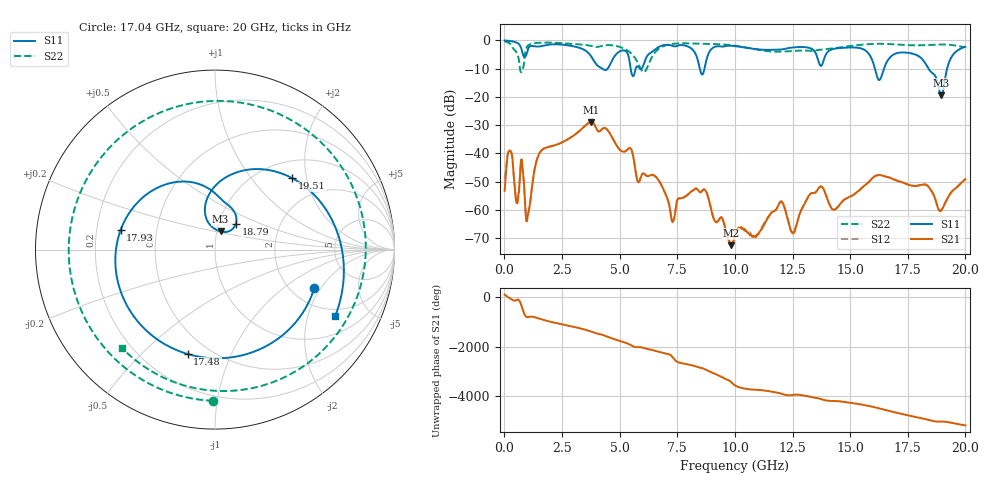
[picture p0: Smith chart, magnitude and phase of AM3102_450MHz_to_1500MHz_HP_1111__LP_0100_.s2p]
!Agilent Technologies,E8364B,MY43040894,A.07.50.67
!Agilent E8364B: A.07.50.67
!Date: Thursday, January 11, 2018 06:49:40
!Correction: S11(Full 2 Port(1,2))
!S21(Full 2 Port(1,2))
!S12(Full 2 Port(1,2))
!S22(Full 2 Port(1,2))
!S2P File: Measurements: S11, S21, S12, S22:
# Hz S  dB  R 50
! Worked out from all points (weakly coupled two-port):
!   1601 points, 10 MHz to 20 GHz, reference 50 ohm
!   highest |S21| = -28.90 dB at 3.758 GHz (marker M1); lowest = -72.5 dB at 9.83 GHz (marker M2)
!   lowest |S11| = -19.5 dB at 18.95 GHz (marker M3), VSWR 1.24, Z = 52.1 + j10.7 ohm
!   |S11| at or under -10 dB: 4.246 GHz to 4.484 GHz (237.6 MHz wide, 5.44 % of centre); 16.07 GHz to 16.47 GHz (396.4 MHz wide, 2.44 % of centre); 18.4 GHz to 19.21 GHz (809.5 MHz wide, 4.31 % of centre)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
!   |S22| runs from -11.3 to -0.3 dB; largest |S21 - S12| = 0.0023
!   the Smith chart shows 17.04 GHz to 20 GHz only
!   S11 on the Smith chart (normalised r, x): 17.04 GHz: 2.65, -1.74; 17.48 GHz: 0.38, -0.70; 17.93 GHz: 0.30, +0.09; 18.79 GHz: 1.20, +0.36; 19.51 GHz: 1.36, +1.65; 20 GHz: 1.68, -3.01
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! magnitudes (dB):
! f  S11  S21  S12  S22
! 10 MHz  -0.1  -53.3  -48.9  -0.3
! 247.4 MHz  -0.3  -39.0  -38.9  -1.2
! 1.01 GHz  -3.6  -62.2  -62.2  -2.0
! 1.547 GHz  -2.1  -39.6  -39.6  -0.9
! 3.346 GHz  -2.9  -31.4  -31.4  -1.5
! 3.758 GHz  -5.6  -28.9  -28.9  -2.0
! 6.682 GHz  -2.4  -49.4  -49.4  -3.1
! 7.306 GHz  -2.0  -64.3  -64.0  -1.3
! 8.706 GHz  -9.1  -53.0  -53.0  -1.3
! 9.83 GHz  -1.9  -72.5  -72.8  -1.7
! 10.01 GHz  -2.1  -68.8  -69.6  -1.9
! 12 GHz  -3.3  -57.0  -57.1  -4.0
! 12.53 GHz  -2.5  -68.1  -68.2  -3.8
! 13.34 GHz  -3.1  -54.1  -54.0  -3.8
! 16.68 GHz  -6.6  -48.5  -48.5  -1.3
! 17.04 GHz  -4.5  -49.7  -49.7  -1.5
! 17.48 GHz  -4.4  -51.0  -51.0  -1.7
! 17.93 GHz  -5.4  -51.5  -51.4  -1.8
! 18.79 GHz  -14.6  -58.9  -58.6  -1.5
! 18.95 GHz  -19.5  -60.2  -60.1  -1.5
! 19.51 GHz  -4.6  -52.8  -52.8  -1.8
! 20 GHz  -2.3  -49.2  -49.2  -2.4
